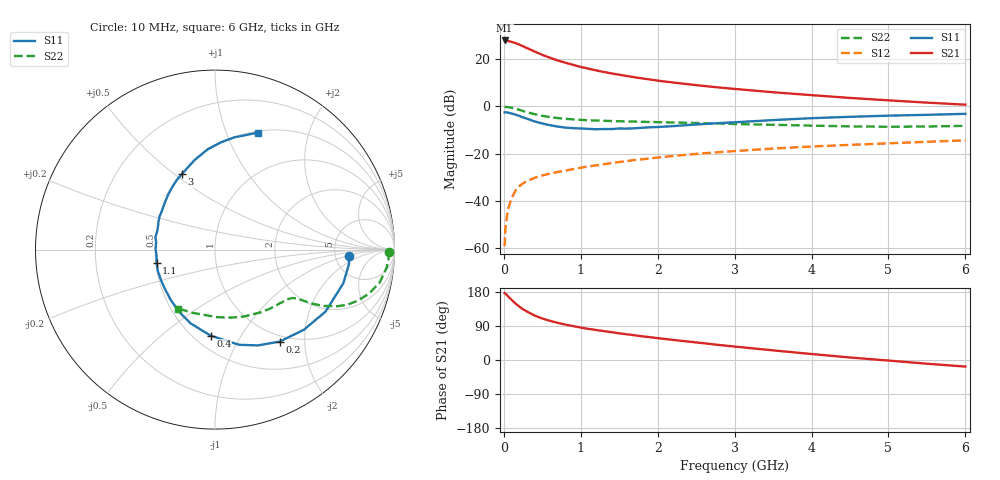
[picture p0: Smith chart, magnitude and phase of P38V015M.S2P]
! SIEMENS Small Signal Semiconductors
! BFP181
! Si NPN RF Bipolar Junction Transistor in SOT143
! VCE = 8 V  IC = 15 mA
! Common Emitter S-Parameters:  March  1996
# GHz  S  MA  R  50
!  f  S11  S21  S12  S22
! GHz  MAG  ANG  MAG  ANG  MAG  ANG  MAG  ANG
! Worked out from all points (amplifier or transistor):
!   36 points, 10 MHz to 6 GHz, reference 50 ohm
!   highest |S21| = 27.9 dB at 10 MHz (marker M1)
!   |S21| within 3 dB of that: start of sweep to 285.4 MHz
!   unconditionally stable (mu >= 1): 1.109 GHz to end of sweep
!   at 250 MHz: K = 0.38, MSG = 29.0 dB, |S12| = -32.6 dB
!   at 1.4 GHz: K = 1.08, MAG = 17.2 dB, |S12| = -24.0 dB
!   at 6 GHz: K = 1.01, MAG = 6.9 dB, |S12| = -14.4 dB
!   S11 on the Smith chart (normalised r, x): 10 MHz: 6.67, -1.13; 200 MHz: 0.91, -1.53; 400 MHz: 0.60, -0.75; 1.1 GHz: 0.50, -0.08; 3 GHz: 0.50, +0.53; 6 GHz: 0.52, +1.29
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0.01  0.7458 -2.9  24.75 176.5  0.0011 81.3  0.972 -0.7
0.02  0.751 -6.0  24.59 175.3  0.0026 84.3  0.9701 -2.1
0.05  0.7392 -14.7  24.28 169.0  0.0063 83.5  0.9628 -5.8
0.1  0.7061 -29.3  23.13 158.9  0.0112 73.8  0.9352 -11.4
0.15  0.6668 -42.0  21.82 149.4  0.0164 70.2  0.8902 -16.1
0.2  0.6267 -54.8  20.32 141.0  0.0204 65.8  0.8437 -19.8
0.25  0.5852 -65.8  18.58 133.8  0.0235 61.6  0.7957 -22.8
0.3  0.5471 -75.8  17.11 128.0  0.0262 59.7  0.7514 -24.8
0.4  0.4801 -92.9  14.42 117.4  0.0307 55.6  0.6821 -27.4
0.5  0.4329 -108.3  12.25 109.5  0.0345 53.2  0.6299 -28.8
0.6  0.3992 -120.4  10.69 103.3  0.0376 52.4  0.5919 -29.6
0.7  0.3731 -131.5  9.319 98.0  0.0408 52.6  0.5649 -30.1
0.9  0.3455 -150.5  7.54 89.5  0.0471 52.3  0.5298 -30.9
1.1  0.3334 -167.4  6.269 82.1  0.0537 52.1  0.5078 -32.1
1.3  0.3313 179.5  5.323 76.1  0.0596 52.1  0.4941 -33.8
1.6  0.3375 162.9  4.379 67.8  0.0695 51.2  0.4798 -36.7
2.2  0.3813 137.5  3.192 53.0  0.0891 48.1  0.4553 -44.5
3  0.4593 113.8  2.337 35.5  0.1131 42.4  0.4229 -57.2
3.5  0.5121 102.8  1.985 25.4  0.1278 38.6  0.4067 -66.4
4.5  0.5997 86.6  1.505 6.6  0.153 30.2  0.3768 -87.8
5.5  0.6615 74.8  1.198 -9.8  0.1778 22.8  0.3746 -110.3
6  0.6935 70.0  1.085 -17.3  0.1906 18.8  0.3867 -121.9
